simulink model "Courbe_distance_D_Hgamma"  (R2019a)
settings: Solver=VariableStepAuto  StartTime=0.0  StopTime=6.283185307  MaxStep=0.001  RelTol=1e-6  SampleTimeConstraint=STIndependent

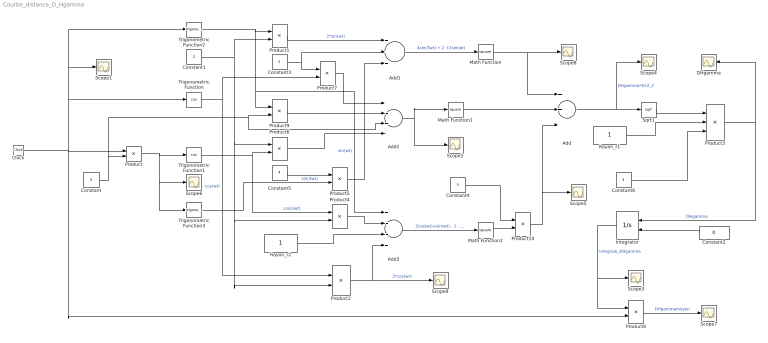
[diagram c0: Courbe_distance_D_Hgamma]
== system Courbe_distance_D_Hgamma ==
  Add : Sum  Inputs=+++
  Add1 : Sum  Inputs=+++
  Add2 : Sum  Inputs=+-+-
  Add3 : Sum  Inputs=+--+
  Clock : Clock
  Constant : Constant  Value=3
  Constant1 : Constant  Value=2
  Constant2 : Constant  Value=0
  Constant3 : Constant  Value=2
  Constant4 : Constant  Value=3
  Constant5 : Constant  Value=4
  Constant6 : Constant  Value=4
  DHgamma : Scope
  Integrator : Integrator  InitialConditionSource=external
  Math Function : Math  Operator=square
  Math Function1 : Math  Operator=square
  Math Function2 : Math  Operator=square
  Product{,1,4..7,9..10} (8 alike) : Product
  Product2 : Product  Inputs=**
  Product3 : Product  Inputs=**/
  Product8 : Product  Inputs=*/
  Rayon_r1 : Constant
  Rayon_r2 : Constant
  Scope{1..9} (9 alike) : Scope
  Sqrt1 : Sqrt
  Trigonometric Function : Trigonometry  Operator=cos
  Trigonometric Function1 : Trigonometry  Operator=cos
  Trigonometric Function2 : Trigonometry
  Trigonometric Function3 : Trigonometry
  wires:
  Product/1 -> Trigonometric Function3/1, Scope6/1, Trigonometric Function1/1
  Clock/1 -> Product8/2, Trigonometric Function/1, Trigonometric Function2/1, Scope1/1, Product/1
  Trigonometric Function2/1 -> Add3/1, Product9/1, Product1/1  "sin(wt)"
  Product1/1 -> Add1/1  "2*sin(wt)"
  Add1/1 -> Math Function/1  "4sin(3wt) + 2 +2sin(wt)"
  Add2/1 -> Math Function1/1, Scope2/1
  Add3/1 -> Math Function2/1  "2cos(wt)+sin(wt) - 1 - 2cos(3wt)"
  Math Function/1 -> Scope8/1, Add/1
  Add/1 -> Sqrt1/1, Scope4/1  "DHgamma*4/r2_2"
  Integrator/1 -> Product8/1, Scope3/1  "Integrale_DHgamma"
  Constant2/1 -> Integrator/2
  Product8/1 -> Scope7/1  "DHgammamoyen"
  Constant1/1 -> Product4/2, Product2/2, Product6/1, Product1/2
  Trigonometric Function3/1 -> Product5/2  "sin(3wt)"
  Constant3/1 -> Product7/1, Add1/2
  Sqrt1/1 -> Product3/1
  Constant6/1 -> Product3/3
  Product3/1 -> Integrator/1, DHgamma/1  "DHgamma"
  Product2/1 -> Add3/4, Scope9/1  "2*cos(wt)"
  Product5/1 -> Add1/3
  Constant5/1 -> Product5/1
  Product6/1 -> Add2/4
  Trigonometric Function1/1 -> Product6/2, Product4/1  "cos(3wt)"
  Constant/1 -> Add2/3, Product9/2, Product/2
  Trigonometric Function/1 -> Product2/1, Product7/2  "cos(wt)"
  Product9/1 -> Add2/2
  Rayon_r1/1 -> Product3/2
  Rayon_r2/1 -> Add3/3
  Product4/1 -> Add3/2
  Math Function2/1 -> Product10/2
  Product10/1 -> Scope5/1, Add/3
  Constant4/1 -> Product10/1
  Math Function1/1 -> Add/2
  Product7/1 -> Add2/1
